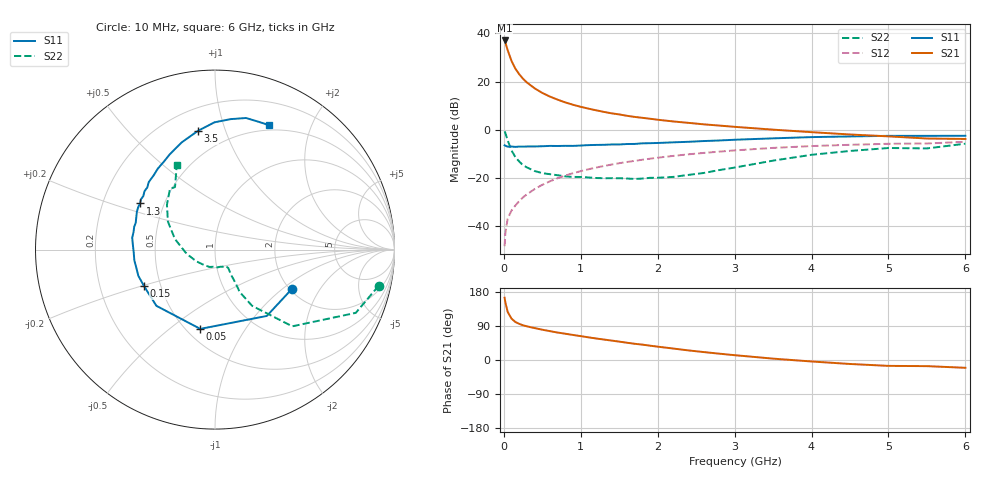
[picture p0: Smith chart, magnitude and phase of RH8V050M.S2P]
! SIEMENS Small Signal Semiconductors
! BFR106
! Si NPN RF Bipolar Junction Transistor in SOT23
! VCE = 8 V  IC = 50 mA
! Common Emitter S-Parameters:  August  1996
# GHz  S  MA  R  50
!  f  S11  S21  S12  S22
! GHz  MAG  ANG  MAG  ANG  MAG  ANG  MAG  ANG
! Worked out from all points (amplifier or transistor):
!   36 points, 10 MHz to 6 GHz, reference 50 ohm
!   highest |S21| = 37.1 dB at 10 MHz (marker M1)
!   |S21| within 3 dB of that: start of sweep to 40.26 MHz
!   unconditionally stable (mu >= 1): 263 MHz to 2.271 GHz
!   at 250 MHz: K = 0.99, MSG = 24.5 dB, |S12| = -27.9 dB
!   at 1.4 GHz: K = 1.06, MAG = 9.1 dB, |S12| = -14.4 dB
!   at 6 GHz: K = 0.98, MSG = 0.6 dB, |S12| = -4.9 dB
!   S11 on the Smith chart (normalised r, x): 10 MHz: 2.05, -1.17; 50 MHz: 0.58, -0.65; 150 MHz: 0.40, -0.21; 1.3 GHz: 0.37, +0.25; 3.5 GHz: 0.34, +0.81; 6 GHz: 0.44, +1.43
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0.01  0.4809 -27.2  71.33 164.3  0.0039 81.6  0.9333 -12.5
0.02  0.4691 -52.0  64.94 151.9  0.0074 73.3  0.8599 -24.2
0.05  0.4493 -100.5  44.75 126.8  0.0145 60.6  0.6066 -44.8
0.1  0.4525 -136.2  26.84 109.1  0.0214 59.3  0.3748 -56.6
0.15  0.4445 -152.6  18.58 100.3  0.0272 62.7  0.273 -59.8
0.2  0.4514 -161.1  14.24 95.4  0.0335 65.9  0.2213 -58.5
0.25  0.4499 -167.3  11.45 91.5  0.0402 68.0  0.1852 -57.9
0.3  0.4534 -172.4  9.601 88.8  0.0463 69.5  0.167 -57.5
0.4  0.4534 -178.6  7.276 84.2  0.0594 70.9  0.1406 -55.6
0.5  0.4589 176.3  5.832 80.0  0.0728 71.3  0.1272 -54.2
0.6  0.4661 171.8  4.894 76.1  0.0863 71.4  0.1208 -55.0
0.7  0.4642 167.8  4.229 72.4  0.0999 70.6  0.115 -56.9
0.9  0.4664 161.3  3.317 66.0  0.1268 68.7  0.1062 -59.8
1.1  0.4839 154.1  2.758 59.8  0.1528 66.5  0.1034 -67.9
1.3  0.491 148.4  2.362 54.0  0.1788 64.0  0.0998 -75.0
1.7  0.5121 137.4  1.859 42.8  0.2284 58.8  0.0963 -96.6
2.2  0.5523 125.2  1.499 30.3  0.289 51.8  0.1062 -127.7
2.8  0.6038 111.5  1.23 16.7  0.355 43.0  0.1471 -166.1
3.5  0.6683 98.2  1.012 3.6  0.424 32.9  0.2309 165.2
4.5  0.732 83.2  0.804 -10.5  0.4911 18.2  0.3661 137.0
5.5  0.7525 70.7  0.663 -16.2  0.5237 8.2  0.4134 122.6
6  0.7558 66.7  0.649 -20.6  0.5661 1.0  0.5174 114.3
